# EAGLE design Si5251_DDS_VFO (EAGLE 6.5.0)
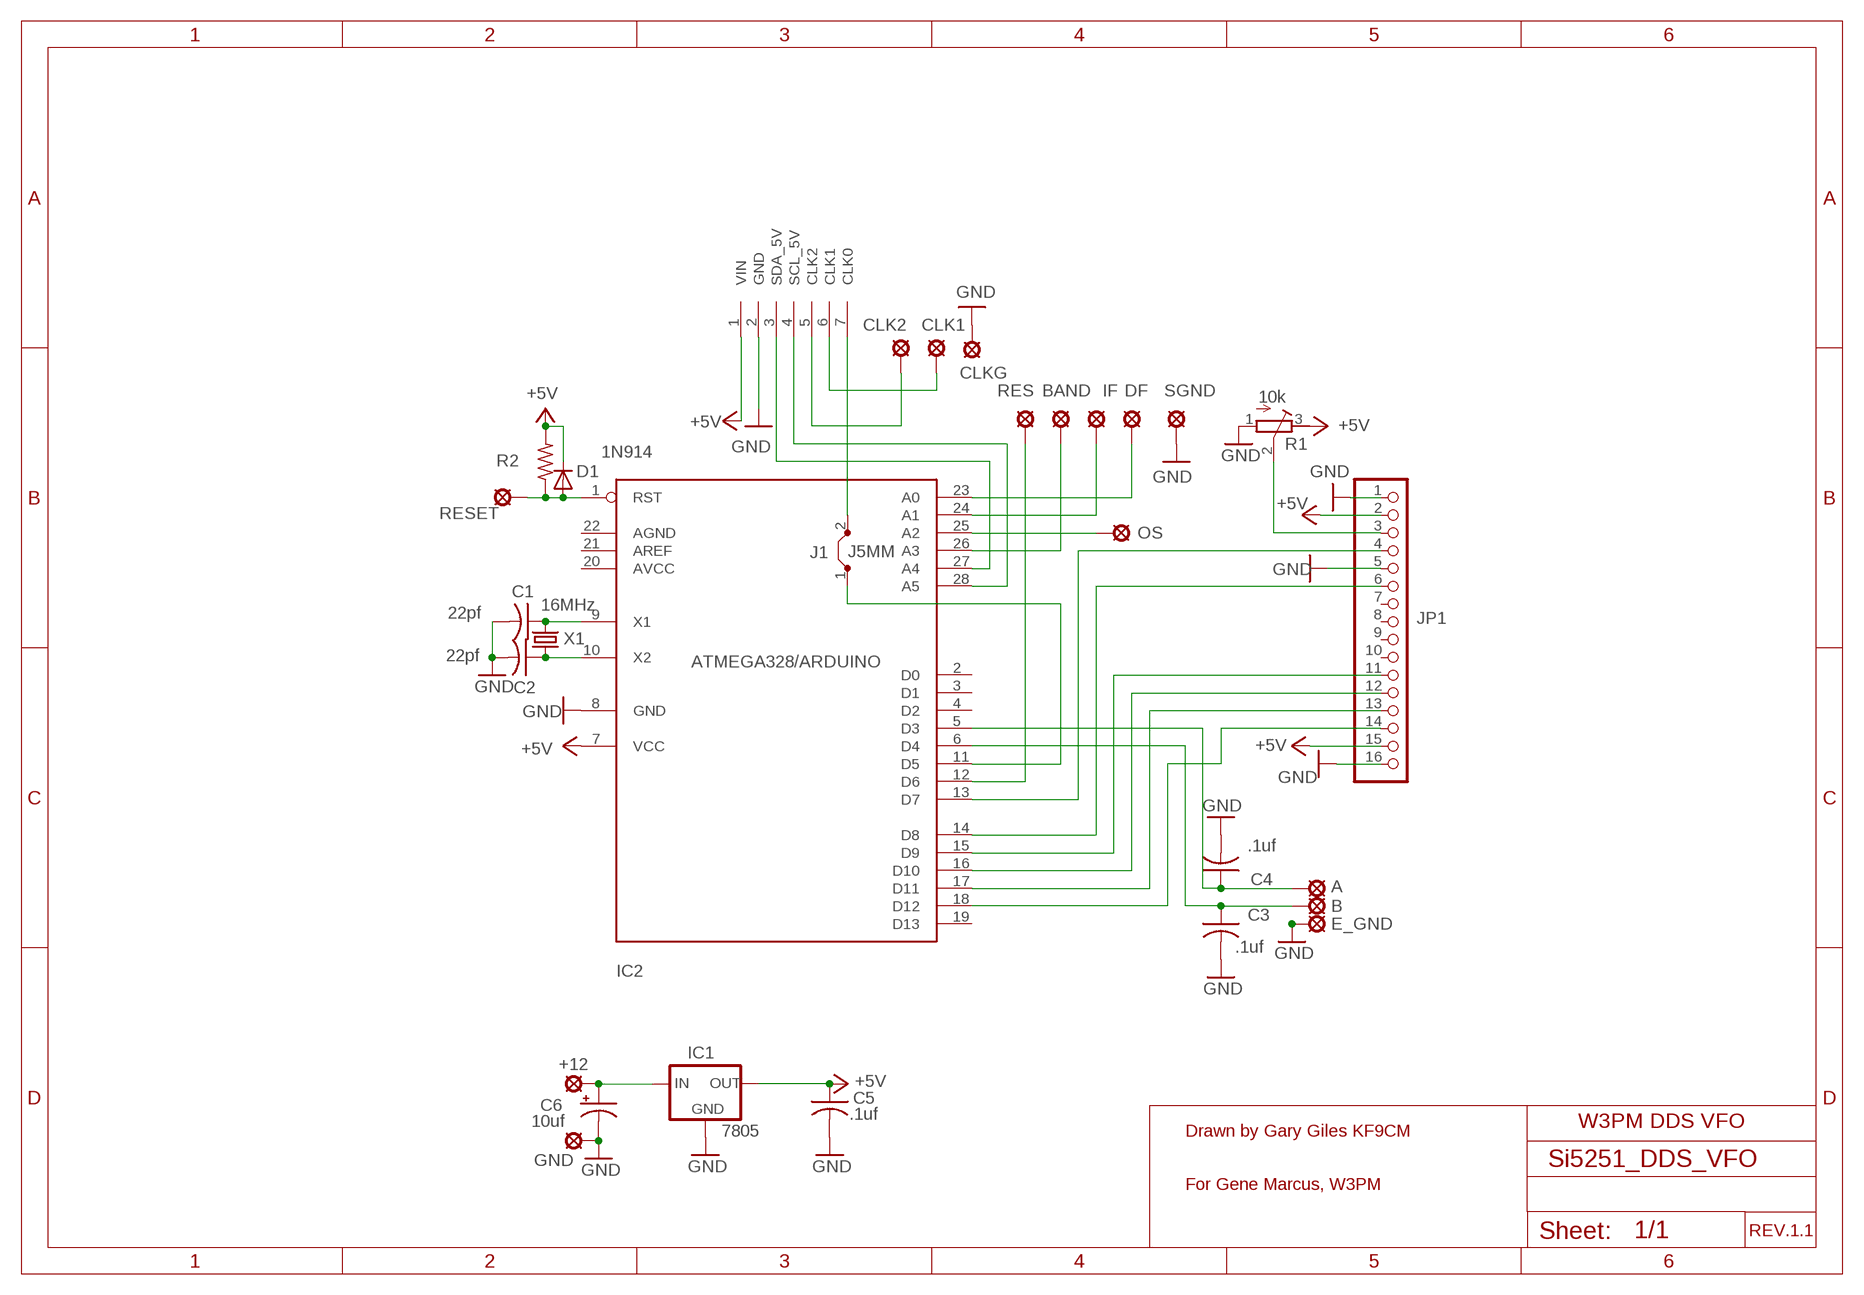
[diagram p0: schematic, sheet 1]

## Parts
+12  LSP10  [LSP10]
A  LSP10  [LSP10]
B  LSP10  [LSP10]
BAND  LSP10  [LSP10]
C1  22pf  C-US025-024X044  [C025-024X044]
C2  22pf  C-US025-024X044  [C025-024X044]
C3  .1uf  C-US025-024X044  [C025-024X044]
C4  .1uf  C-US025-024X044  [C025-024X044]
C5  .1uf  C-US025-024X044  [C025-024X044]
C6  10uf  CPOL-USE2.5-6  [E2,5-6]
CLK1  LSP10  [LSP10]
CLK2  LSP10  [LSP10]
CLKG  LSP10  [LSP10]
D1  1N914  1N914TS  [DIODETS]
DF  LSP10  [LSP10]
E_GND  LSP10  [LSP10]
GND  LSP10  [LSP10]
IC1  7805  78XXS  [78XXS]
IC2  ATMEGA328/ARDUINO  [DIL28-3]
IF  LSP10  [LSP10]
J1  J5MM  [05]
JP1  PINHD-1X16  [1X16]
OS  LSP10  [LSP10]
R1  10k  R-TRIMM3339P  [RTRIM3339P]
R2  R-US_0204/2V  [0204V]
RES  LSP10  [LSP10]
RESET  LSP10  [LSP10]
SGND  LSP10  [LSP10]
U$1  SI5351  [SI5351]
X1  16MHz  CRYTALHC49U-V  [HC49U-V]

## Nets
+5V: C5.1 D1.2(C) IC1.OUT IC2.7(VCC) JP1.2 JP1.15 R1.3(E) R2.2 U$1.1(VIN)
GND: C1.2 C2.2 C3.2 C4.2 C5.2 C6.- CLKG.MP E_GND.MP GND.MP IC1.GND IC2.8(GND) JP1.1 JP1.5 JP1.16 R1.1(A) SGND.MP U$1.2(GND)
N$1: D1.1(A) IC2.1(RST) R2.1 RESET.MP
N$2: IC2.13(D7) JP1.4
N$3: IC2.14(D8) JP1.6
N$4: IC2.15(D9) JP1.11
N$5: IC2.16(D10) JP1.12
N$6: IC2.17(D11) JP1.13
N$7: JP1.3 R1.2(S)
N$8: IC2.18(D12) JP1.14
N$9: IC2.12(D6) RES.MP
N$10: BAND.MP IC2.26(A3)
N$11: IC2.24(A1) IF.MP
N$13: DF.MP IC2.23(A0)
N$14: A.MP C4.1 IC2.5(D3)
N$15: B.MP C3.1 IC2.6(D4)
N$17: C1.1 IC2.9(X1) X1.2
N$18: C2.1 IC2.10(X2) X1.1
N$19: +12.MP C6.+ IC1.IN
N$20: IC2.27(A4) U$1.3(SDA_5V)
N$21: IC2.28(A5) U$1.4(SCL_5V)
N$53: IC2.25(A2) OS.MP
N$54: J1.2 U$1.7(CLK0)
N$63: IC2.11(D5) J1.1
N$64: CLK2.MP U$1.5(CLK2)
N$65: CLK1.MP U$1.6(CLK1)
Unconnected: IC2.2(D0) IC2.3(D1) IC2.4(D2) IC2.19(D13) IC2.20(AVCC) IC2.21(AREF) IC2.22(AGND) JP1.7 JP1.8 JP1.9 JP1.10

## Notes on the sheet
- W3PM DDS VFO
- Drawn by Gary Giles KF9CM
- For Gene Marcus, W3PM
- REV.1.1

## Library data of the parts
+12 A B BAND CLK1 CLK2 CLKG DF E_GND GND IF OS RES RESET SGND = solpad:LSP10: SOLDER PAD
C1-C5 = 0HamRadio:C-US: CAPACITOR, American symbol
C6 = 0HamRadio:CPOL-US: POLARIZED CAPACITOR, American symbol
D1 = 0HamRadio:1N914TS
IC1 = v-reg:78XXS: VOLTAGE REGULATOR
IC2 = adafruit:ATMEGA328/ARDUINO
J1 = 0HamRadio:J: Bridge
JP1 = pinhead:PINHD-1X16: PIN HEADER
R1 = 0HamRadio:R-TRIMM: Trimm resistor
R2 = 0HamRadio:R-US_: RESISTOR, American symbol
U$1 = 1arduino_build:SI5351
X1 = 0HamRadio:CRYTAL: CRYSTAL

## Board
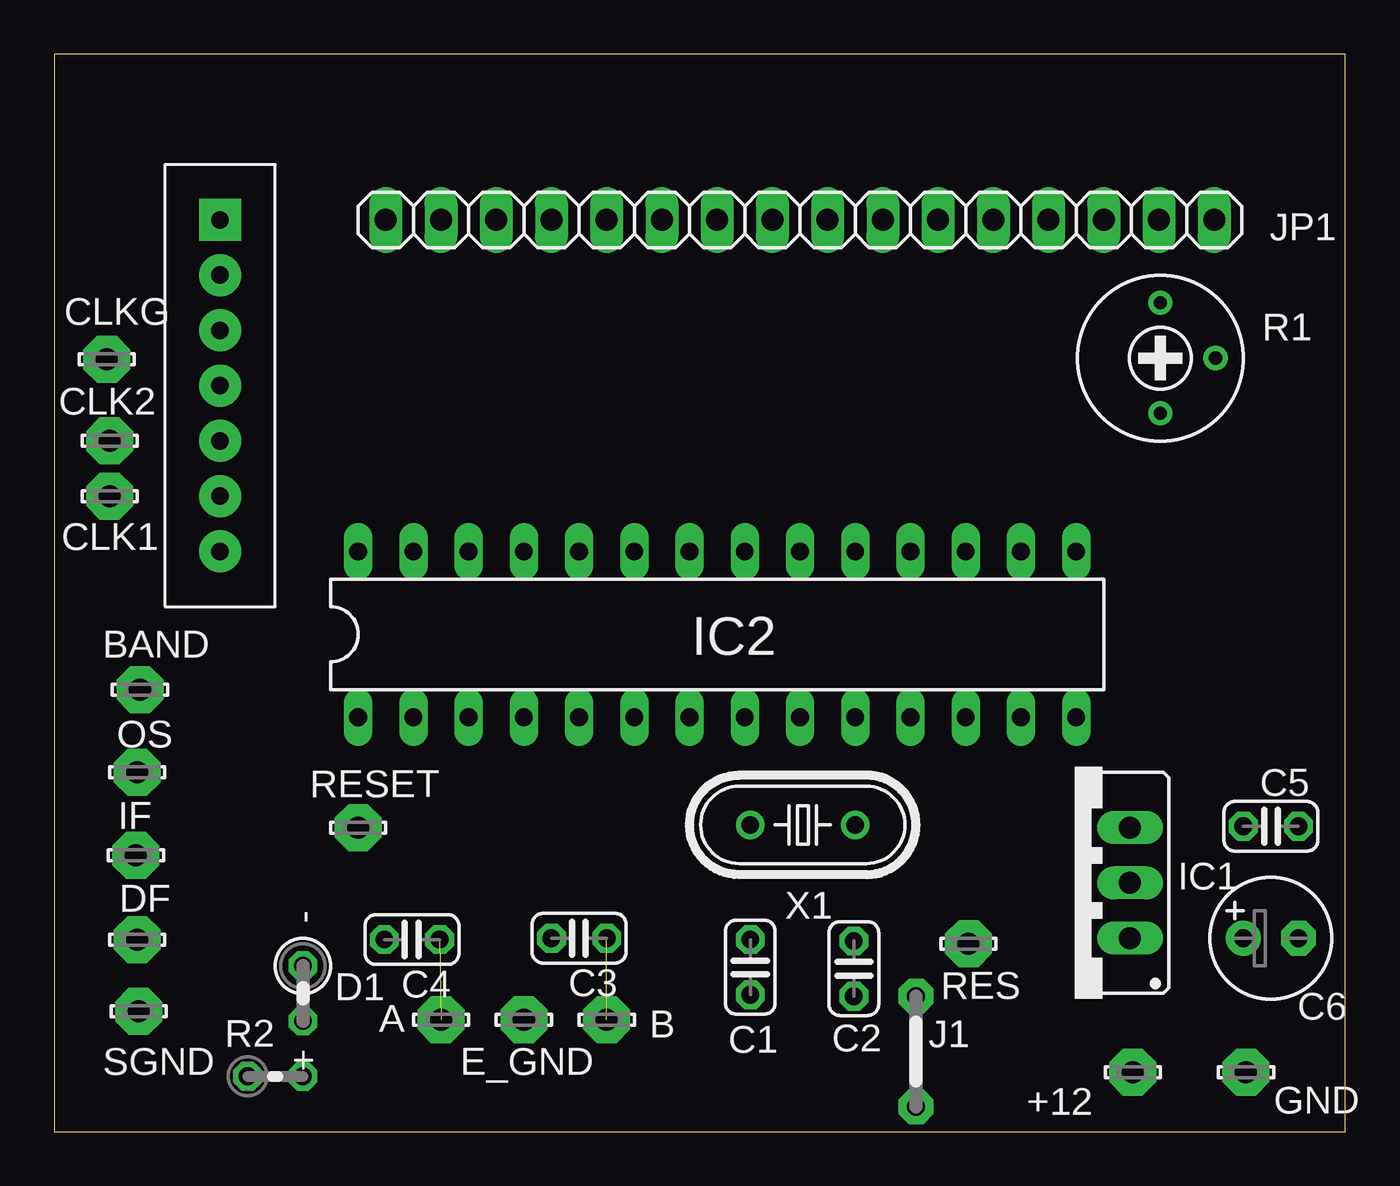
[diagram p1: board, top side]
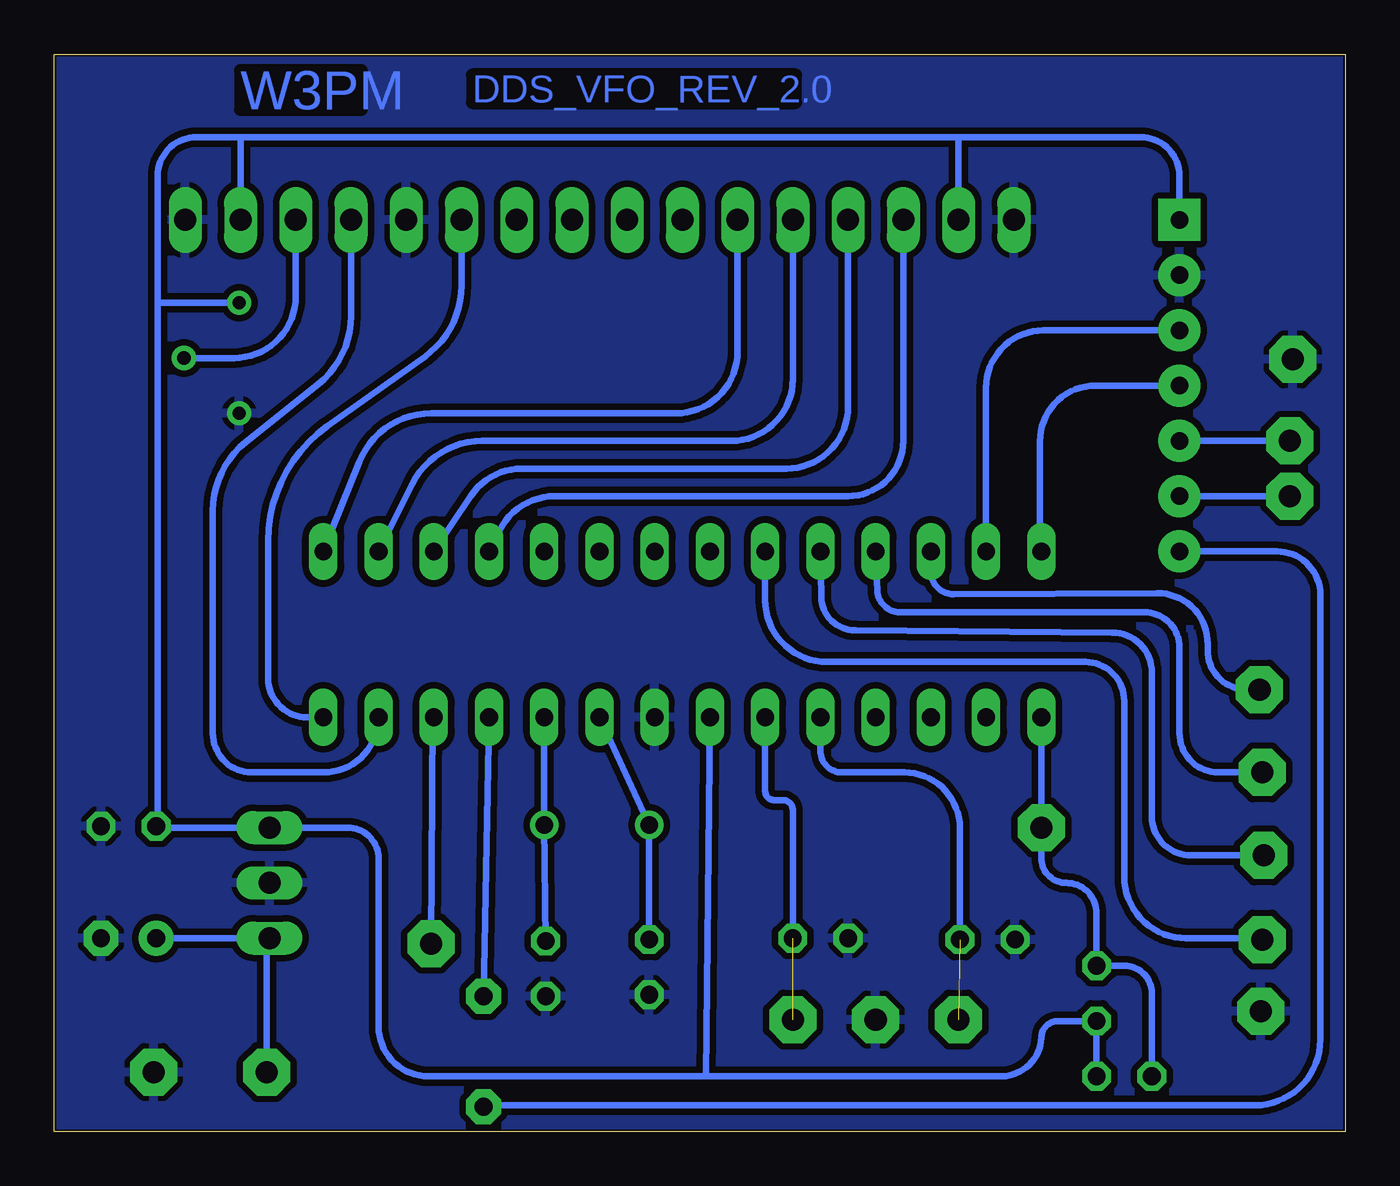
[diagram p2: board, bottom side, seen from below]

Size 59.36 x 49.52 mm. Coordinates in mm from the lower left corner, seen from the top.
Outline: 0,0 59.36,0 59.36,49.52 0,49.52 0,0
Copper layers (1*16): Top 0.035mm / dielectric 1.5mm / Bottom 0.035mm
Design rules "default *": minimum track width 0.3mm, minimum drill 24mil, track to track 0.3mm, track to pad 0.3mm, pad to pad 8mil, via to via 8mil, smd to smd 8mil, copper to edge 0.1mm, drill to drill 8mil, minimum pad ring 10mil, minimum via ring 8mil, stop-mask expansion 4mil, vias tented up to drill 0mil, thermal gap 10mil

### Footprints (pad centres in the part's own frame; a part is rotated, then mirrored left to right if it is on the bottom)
LSP10 = drill 1.016 pad 2.159 octagon: MP 0,0
C025-024X044 = drill 0.813 octagon: 1 -1.27,0; 2 1.27,0
E2,5-6 = drill 0.813 pad 1.6: + -1.27,0 | drill 0.813 pad 1.6 octagon: - 1.27,0
DIODETS = drill 0.813 octagon: 1 -1.27,0; 2 1.27,0
78XXS = drill 1.016 long: GND 0,-2.54; IN -2.54,-2.54; OUT 2.54,-2.54
DIL28-3 = drill 0.813 long: 1 -16.51,-3.81; 2 -13.97,-3.81; 3 -11.43,-3.81; 4 -8.89,-3.81; 5 -6.35,-3.81; 6 -3.81,-3.81; 7 -1.27,-3.81; 8 1.27,-3.81; 9 3.81,-3.81; 10 6.35,-3.81; 11 8.89,-3.81; 12 11.43,-3.81; 13 13.97,-3.81; 14 16.51,-3.81; 15 16.51,3.81; 16 13.97,3.81; 17 11.43,3.81; 18 8.89,3.81; 19 6.35,3.81; 20 3.81,3.81; 21 1.27,3.81; 22 -1.27,3.81; 23 -3.81,3.81; 24 -6.35,3.81; 25 -8.89,3.81; 26 -11.43,3.81; 27 -13.97,3.81; 28 -16.51,3.81
05 = drill 0.813 pad 1.6 octagon: 1 -2.54,0; 2 2.54,0
1X16 = drill 1.016 long: 1 -19.05,0; 2 -16.51,0; 3 -13.97,0; 4 -11.43,0; 5 -8.89,0; 6 -6.35,0; 7 -3.81,0; 8 -1.27,0; 9 1.27,0; 10 3.81,0; 11 6.35,0; 12 8.89,0; 13 11.43,0; 14 13.97,0; 15 16.51,0; 16 19.05,0
RTRIM3339P = drill 0.61: 1 -2.54,0; 2 0,-2.54; 3 2.54,0
0204V = drill 0.813 octagon: 1 -1.27,0; 2 1.27,0
SI5351 = drill 0.8 pad 1.93 square: 1 -1.27,7.62 | drill 0.8 pad 1.93: 2 -1.27,5.08; 3 -1.27,2.54; 4 -1.27,0; 5 -1.27,-2.54; 6 -1.27,-5.08; 7 -1.27,-7.62
HC49U-V = drill 0.813: 1 -2.413,0; 2 2.413,0

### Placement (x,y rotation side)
+12  49.59,2.73 0 top
A  17.78,5.14 0 top
B  25.4,5.14 0 top
BAND  3.94,20.32 0 top
C1  32,7.56 270 top
C2  36.77,7.49 270 top
C3  24.13,8.89 180 top
C4  16.45,8.83 180 top
C5  55.94,14.03 0 top
C6  55.94,8.89 0 top
CLK1  2.54,29.21 0 top
CLK2  2.54,31.75 0 top
CLKG  2.41,35.5 0 top
D1  11.43,6.35 270 top
DF  3.81,8.83 0 top
E_GND  21.59,5.14 0 top
GND  54.8,2.73 0 top
IC1  46.93,11.43 90 top
IC2  30.48,22.86 0 top
IF  3.75,12.7 0 top
J1  39.62,3.68 270 top
JP1  34.29,41.91 180 top
OS  3.81,16.51 0 top
R1  50.86,35.56 90 top
R2  10.16,2.54 0 top
RES  42.04,8.64 0 top
RESET  13.97,13.97 0 top
SGND  3.87,5.52 0 top
U$1  8.89,34.29 0 top
X1  34.42,14.1 180 top

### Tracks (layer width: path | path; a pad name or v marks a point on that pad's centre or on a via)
+5V
  Bottom 0.3: U$1.1 7.62,43.92 arc-90 9.42,45.72 17.78,45.72 | 17.78,45.72 50.8,45.72 | 50.8,45.72 JP1.2 | JP1.15 17.78,45.72 | 54.61,38.1 54.61,14.03 C5.1 54.67,13.97 IC1.OUT 45.88,13.97 arc90 44.45,12.54 44.45,4.83 arc-90 42.16,2.54 29.4,2.54 | 54.61,38.1 54.61,43.92 arc90 52.81,45.72 50.8,45.72 | R1.3 54.61,38.1 | R2.2 D1.2 13.21,5.08 arc-90 13.97,4.32 arc90 15.94,2.54 29.4,2.54 | IC2.7 29.4,2.54
GND
  pour Bottom: 0,49.53 0,0 59.69,0 59.69,49.53
N$1
  Bottom 0.3: IC2.1 RESET.MP 13.97,12.57 arc-90 12.83,11.43 arc90 11.43,10.03 D1.1 10.16,7.62 arc90 8.89,6.35 R2.1
N$2
  Bottom 0.3: JP1.4 45.72,37.49 arc51 47.23,34.35 50.56,31.69 arc-51 52.07,28.55 52.07,18.31 arc-90 50.27,16.51 46.99,16.51 arc-90 IC2.13
N$3
  Bottom 0.3: IC2.14 47.73,19.05 arc90 49.53,20.85 49.53,27.15 arc54 46.82,32.42 42.32,35.63 arc-54 40.64,38.9 JP1.6
N$4
  Bottom 0.3: IC2.15 45.35,30.76 arc68 42.02,33.02 30.78,33.02 arc-90 27.94,35.86 JP1.11
N$5
  Bottom 0.3: IC2.16 42.9,29.76 arc63 39.69,31.75 28.24,31.75 arc-90 25.4,34.59 JP1.12
N$6
  Bottom 0.3: IC2.17 40.21,29.21 arc56 37.85,30.48 25.7,30.48 arc-90 22.86,33.32 JP1.13
N$7
  Bottom 0.3: R1.2 51.1,35.56 arc-90 48.26,38.4 JP1.3
N$8
  Bottom 0.3: IC2.18 38.88,27.64 arc63 36.34,29.21 22.86,29.21 arc-90 20.32,31.75 JP1.14
N$9
  Bottom 0.3: IC2.12 41.97,19.05 RES.MP
N$10
  Bottom 0.3: IC2.26 19.05,25.74 arc-90 18.01,24.71 8.66,24.75 arc91 6.32,22.39 6.32,22.14 arc-91 4.53,20.32 BAND.MP
N$11
  Bottom 0.3: IC2.24 24.09,24.59 arc-89 22.53,23.04 10.72,22.94 arc90 8.89,21.1 8.89,14.5 arc-90 7.09,12.7 IF.MP
N$13
  Bottom 0.3: IC2.23 26.67,24.43 arc-90 23.83,21.59 11.96,21.59 arc90 10.16,19.79 10.16,11.73 arc-90 7.32,8.89 3.81,8.89 DF.MP
N$14  (1 unrouted)
  Bottom 0.3: IC2.5 24.13,17.5 arc-90 23.14,16.51 20.28,16.51 arc90 17.72,13.95 C4.1
N$15  (1 unrouted)
  Bottom 0.3: IC2.6 26.67,15.65 arc-90 26.26,15.24 25.86,15.24 arc90 25.4,14.78 C3.1
N$17
  Bottom 0.3: C1.1 X1.2 IC2.9
N$18
  Bottom 0.3: IC2.10 X1.1 C2.1
N$19
  Bottom 0.3: IC1.IN 49.59,8.89 | 49.59,8.89 +12.MP | 49.59,8.89 C6.+
N$20
  Bottom 0.3: IC2.27 16.51,34.2 arc90 13.88,36.83 U$1.3
N$21
  Bottom 0.3: IC2.28 14.03,26.67 14.03,31.74 arc90 11.48,34.29 U$1.4
N$53
  Bottom 0.3: IC2.25 21.51,24.86 arc-87 20.48,23.88 9.25,23.88 arc90 7.62,22.25 7.62,18.31 arc-90 5.82,16.51 OS.MP
N$54
  Bottom 0.3: U$1.7 3.14,26.67 arc90 1.14,24.68 1.14,4.22 arc90 4.16,1.21 39.62,1.21 J1.2
N$63
  Bottom 0.3: IC2.11 J1.1
N$64
  Bottom 0.3: U$1.5 CLK2.MP
N$65
  Bottom 0.3: U$1.6 CLK1.MP

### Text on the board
Bottom: DDS_VFO_REV_2.0 | W3PM | W3PM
